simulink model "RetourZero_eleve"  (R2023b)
settings: Solver=VariableStepAuto  StartTime=0.0  StopTime=10.0  RelTol=1e-3
libraries: fl_lib x22, nesl_utility x5, ee_lib x2

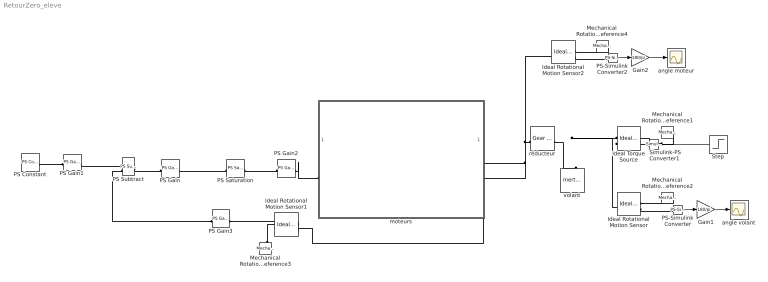
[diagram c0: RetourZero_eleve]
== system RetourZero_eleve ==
  Gain1 : Gain  Gain=180/pi
  Gain2 : Gain  Gain=180/pi
  Ideal Rotational Motion Sensor : fl_lib/Mechanical/Mechanical Sensors/Ideal Rotational Motion Sensor  reference=foundation.enum.MeasurementReference.difference  acceleration_port=false  velocity_port=false  position_port=true  wrap_angle=false  offset=0 rad
  Ideal Rotational Motion Sensor1 : fl_lib/Mechanical/Mechanical Sensors/Ideal Rotational Motion Sensor  reference=foundation.enum.MeasurementReference.difference  acceleration_port=false  velocity_port=false  position_port=true  wrap_angle=false  offset=0 rad
  Ideal Rotational Motion Sensor2 : fl_lib/Mechanical/Mechanical Sensors/Ideal Rotational Motion Sensor  reference=foundation.enum.MeasurementReference.difference  acceleration_port=false  velocity_port=false  position_port=true  wrap_angle=false  offset=0 rad
  Ideal Torque Source : fl_lib/Mechanical/Mechanical Sources/Ideal Torque Source
  Mechanical Rotational Reference{1..4} (4 alike) : fl_lib/Mechanical/Rotational Elements/Mechanical Rotational Reference
  PS Constant : fl_lib/Physical Signals/Sources/PS Constant  constant=0
  PS Gain : fl_lib/Physical Signals/Functions/PS Gain  gain=7
  PS Gain1 : fl_lib/Physical Signals/Functions/PS Gain  gain=120*11/(2*pi*180)
  PS Gain2 : fl_lib/Physical Signals/Functions/PS Gain  gain=24/1204
  PS Gain3 : fl_lib/Physical Signals/Functions/PS Gain  gain=120/(2*pi)
  PS Saturation : fl_lib/Physical Signals/Nonlinear Operators/PS Saturation  upper_limit=1024  lower_limit=-1024
  PS Subtract : fl_lib/Physical Signals/Functions/PS Subtract
  PS-Simulink Converter : nesl_utility/PS-Simulink Converter  PhysicalDomain=network_engine_domain  SubClassName=ps_output  LeftPortType=input  RightPortType=output  PseudoPeriodic=off  Frequencies=[]  VectorFormat=inherit  Unit=inherit  AffineConversion=off
  PS-Simulink Converter2 : nesl_utility/PS-Simulink Converter  PhysicalDomain=network_engine_domain  SubClassName=ps_output  LeftPortType=input  RightPortType=output  PseudoPeriodic=off  Frequencies=[]  VectorFormat=inherit  Unit=inherit  AffineConversion=off
  Simulink-PS Converter1 : nesl_utility/Simulink-PS Converter  PhysicalDomain=network_engine_domain  SubClassName=ps_input  LeftPortType=input  RightPortType=output  PseudoPeriodic=off  Frequencies=[]  NoiseDistribution=none  NoiseParameters=[]  Unit=1  AffineConversion=off  FilteringAndDerivatives=provide  SimscapeFilterOrder=1  InputFilterTimeConstant=0.001  UdotUserProvided=0
  Step : Step  Time=0.3  Before=7  After=0  SampleTime=0
  angle moteur : Scope
  angle volant : Scope
  moteurs : Subsystem  mask{Ke=0, L=0, R=0}
  réducteur : fl_lib/Mechanical/Mechanisms/Gear Box  ratio=0  t_in_specify=off  t_in_priority=None  t_in=0 N*m  t_in_nominal_specify=off  t_in_nominal_unit=N*m  t_in_nominal_value=1  t_out_specify=off  t_out_priority=None  t_out=0 N*m  t_out_nominal_specify=off  t_out_nominal_unit=N*m  t_out_nominal_value=1
  volant : fl_lib/Mechanical/Rotational Elements/Inertia  inertia=0.011 kg*m^2  num_ports=foundation.enum.numPorts2.one  w_specify=off  w_priority=High  w=0 rad/s  w_nominal_specify=off  w_nominal_unit=rad/s  w_nominal_value=1  t_specify=off  t_priority=None  t=0 N*m  t_nominal_specify=off  t_nominal_unit=N*m  t_nominal_value=1
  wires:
  Step/1 -> Simulink-PS Converter1/1
  Gain1/1 -> angle volant/1
  PS-Simulink Converter/1 -> Gain1/1
  PS-Simulink Converter2/1 -> Gain2/1
  Gain2/1 -> angle moteur/1
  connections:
  réducteur/RConn1 -- Ideal Rotational Motion Sensor/LConn1 -- Ideal Torque Source/LConn1 -- volant/LConn1
  Mechanical Rotational Reference1/LConn1 -- Ideal Torque Source/RConn2
  Simulink-PS Converter1/RConn1 -- Ideal Torque Source/RConn1
  Ideal Rotational Motion Sensor/RConn2 -- PS-Simulink Converter/LConn1
  Mechanical Rotational Reference2/LConn1 -- Ideal Rotational Motion Sensor/RConn1
  Mechanical Rotational Reference3/LConn1 -- Ideal Rotational Motion Sensor1/RConn1
  Ideal Rotational Motion Sensor1/RConn2 -- PS Gain3/LConn1
  Mechanical Rotational Reference4/LConn1 -- Ideal Rotational Motion Sensor2/RConn1
  Ideal Rotational Motion Sensor2/RConn2 -- PS-Simulink Converter2/LConn1
  PS Gain/RConn1 -- PS Saturation/LConn1
  PS Saturation/RConn1 -- PS Gain2/LConn1
  PS Constant/RConn1 -- PS Gain1/LConn1
  PS Gain1/RConn1 -- PS Subtract/LConn1
  PS Subtract/RConn1 -- PS Gain/LConn1
  PS Subtract/LConn2 -- PS Gain3/RConn1
  réducteur/LConn1 -- Ideal Rotational Motion Sensor2/LConn1 -- Ideal Rotational Motion Sensor1/LConn1 -- moteurs/LConn1
  PS Gain2/RConn1 -- moteurs/RConn1

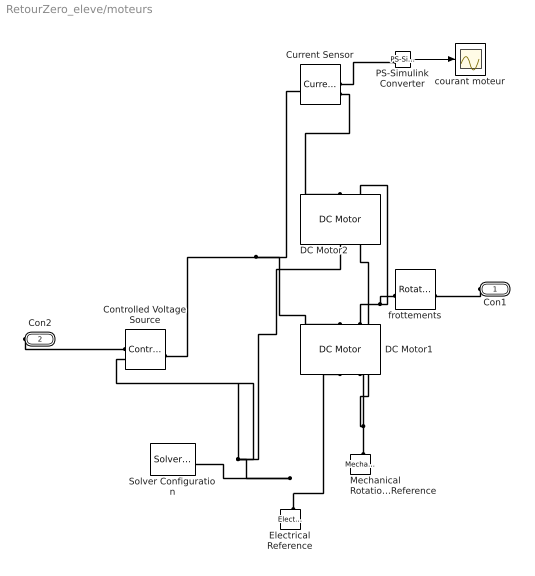
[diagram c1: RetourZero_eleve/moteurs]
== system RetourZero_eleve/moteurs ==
  Controlled Voltage Source : fl_lib/Electrical/Electrical Sources/Controlled Voltage Source
  Current Sensor : fl_lib/Electrical/Electrical Sensors/Current Sensor
  DC Motor1 : ee_lib/Electromechanical/Brushed Motors/DC Motor  field_option=ee.enum.field_option.pm  Rf=100 Ohm  Lf=1 H  Laf=0.15 H  If0=0 A  parameterization=ee.enum.dcparam_option.circuit_param  Ra=R Ohm  La=L H  emf_or_torque=ee.enum.emf_or_torque.ki  Kv=0.072e-3 V*s/rad  Ki=Ke N*m/A  T_stall=0.24e-3 N*m  w_max=19100 rpm  w_rated=15000 rpm  P_rated=0.08 W  V_rated=1.5 V  lam_param=ee.enum.lam_param.damping  i_noload=0 A  V_i_noload=1.5 V  J=2.5e-5 kg*m^2  lam=0 N*m*s/rad  speed0=0 rpm  enable_fault_armature=simscape.enum.onoff.off  rev_faulted=1 / 3  G_faulted_armature=1e-5 S  fault_trigger_armature=ee.enum.faults.faultTrigger.temporal  t_fault_armature=1 s  max_permissible_current_armature=inf A  t_fail_on_current_armature=1 s  enable_fault_field=simscape.enum.onoff.off  G_faulted_field=1e-5 S  fault_trigger_field=ee.enum.faults.faultTrigger.temporal  t_fault_field=1 s  max_permissible_current_field=inf A  t_fail_on_current_field=1 s  fault_action=simscape.enum.assert.action.none  alpha=3.93e-3 1/K  Tmeas=25 degC  thermal_mass=100 J/K  initial_temperature=25 degC
  DC Motor2 : ee_lib/Electromechanical/Brushed Motors/DC Motor  field_option=ee.enum.field_option.pm  Rf=100 Ohm  Lf=1 H  Laf=0.15 H  If0=0 A  parameterization=ee.enum.dcparam_option.circuit_param  Ra=R Ohm  La=L H  emf_or_torque=ee.enum.emf_or_torque.ki  Kv=0.072e-3 V*s/rad  Ki=Ke N*m/A  T_stall=0.24e-3 N*m  w_max=19100 rpm  w_rated=15000 rpm  P_rated=0.08 W  V_rated=1.5 V  lam_param=ee.enum.lam_param.damping  i_noload=0 A  V_i_noload=1.5 V  J=2.5e-5 kg*m^2  lam=0 N*m*s/rad  speed0=0 rpm  enable_fault_armature=simscape.enum.onoff.off  rev_faulted=1 / 3  G_faulted_armature=1e-5 S  fault_trigger_armature=ee.enum.faults.faultTrigger.temporal  t_fault_armature=1 s  max_permissible_current_armature=inf A  t_fail_on_current_armature=1 s  enable_fault_field=simscape.enum.onoff.off  G_faulted_field=1e-5 S  fault_trigger_field=ee.enum.faults.faultTrigger.temporal  t_fault_field=1 s  max_permissible_current_field=inf A  t_fail_on_current_field=1 s  fault_action=simscape.enum.assert.action.none  alpha=3.93e-3 1/K  Tmeas=25 degC  thermal_mass=100 J/K  initial_temperature=25 degC
  Electrical Reference : fl_lib/Electrical/Electrical Elements/Electrical Reference
  Mechanical Rotational Reference : fl_lib/Mechanical/Rotational Elements/Mechanical Rotational Reference
  PS-Simulink Converter : nesl_utility/PS-Simulink Converter  PhysicalDomain=network_engine_domain  SubClassName=ps_output  LeftPortType=input  RightPortType=output  PseudoPeriodic=off  Frequencies=[]  VectorFormat=inherit  Unit=inherit  AffineConversion=off
  Solver Configuration : nesl_utility/Solver Configuration  PhysicalDomain=network_engine_domain  SubClassName=solver  LeftPortType=input  RightPortType=generic  Tones=[]  Harmonics=[]  SimulateNoise=off  Profile=off  UseLocalSampling=off  EnableSwitchedLinearOptims=on  FrequencyDomain=off  UseCCode=off  RelTol=0.001  AbsTol=0.001  MinStep=1e-09  ToWorkspace=off  RevertToSquareIcSolve=off  NumHomotopyIterations=100  PhasorMode=off  PhasorModeNumHarmonics=1  ConsistencySolver=NEWTON_XTOL_AFTER_FTOL  IndexReductionMethod=DerivativeReplacement  DoDC=off  ResidualTolerance=1e-09  ConsistencyTolSource=GLOBAL  ConsistencyAbsTol=0.001  ConsistencyRelTol=0.001  ConsistencyTolFactor=0.001  UseLocalSolver=on  LocalSolverChoice=NE_BACKWARD_EULER_ADVANCER  ResolveIndetEquations=on  FunctionEvalNumThread=1  LocalSolverSampleTime=0.001  DoFixedCost=on  MaxNonlinIter=3  MaxModeIter=2  ComputeImpulses=off  ImpulseIterations=2  LinearAlgebra=auto  LinearAlgebraNumThread=0  EquationFormulation=NE_TIME_EF  DelaysMemoryBudget=1024  AutomaticFiltering=on  FilteringTimeConstant=0.001  PartitionStorageMethod=AS_NEEDED  PartitionMemoryBudget=1024  PartitionMethod=ROBUST  MultibodyUseLocalSolver=on  MultibodyLocalSolverChoice=ODE1  MultibodyLocalSolverSampleTime=0.001
  courant moteur : Scope
  frottements : fl_lib/Mechanical/Rotational Elements/Rotational Friction  brkwy_trq=1 N*m  brkwy_vel=0.1 rad/s  Col_trq=16e-3 N*m  visc_coef=0.001 N*m*s/rad  w_specify=off  w_priority=None  w=0 rad/s  w_nominal_specify=off  w_nominal_unit=rad/s  w_nominal_value=1  t_specify=off  t_priority=None  t=0 N*m  t_nominal_specify=off  t_nominal_unit=N*m  t_nominal_value=1
  Con1 : PMIOPort  Side=Left
  Con2 : PMIOPort  Port=2  Side=Right
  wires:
  PS-Simulink Converter/1 -> courant moteur/1
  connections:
  Con1/RConn1 -- frottements/RConn1
  Electrical Reference/LConn1 -- Controlled Voltage Source/RConn2 -- DC Motor2/RConn1 -- Solver Configuration/RConn1 -- DC Motor1/RConn1
  Mechanical Rotational Reference/LConn1 -- DC Motor2/RConn2 -- DC Motor1/RConn2
  Controlled Voltage Source/LConn1 -- Current Sensor/LConn1 -- DC Motor1/LConn1
  Con2/RConn1 -- Controlled Voltage Source/RConn1
  DC Motor1/LConn2 -- DC Motor2/LConn2 -- frottements/LConn1
  Current Sensor/RConn2 -- DC Motor2/LConn1
  Current Sensor/RConn1 -- PS-Simulink Converter/LConn1
